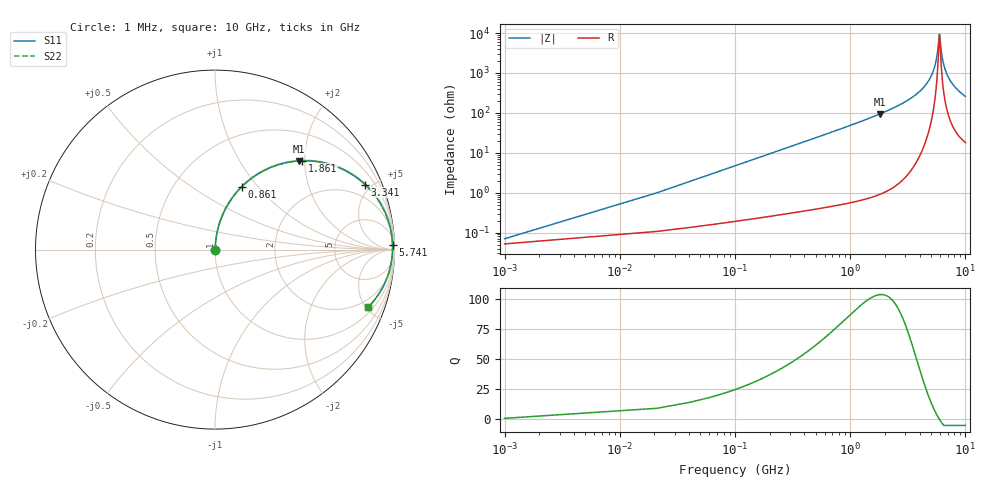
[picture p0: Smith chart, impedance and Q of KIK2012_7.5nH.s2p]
!version-2
!date-01.2022
!Series
# MHz S RI R 50
!Freq ReS11 ImS11 ReS21 ImS21 ReS12 ImS12 ReS22 ImS22
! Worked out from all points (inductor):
!   501 points, 1 MHz to 10 GHz, reference 50 ohm
!   read as one part in series: L = 7.5 nH near 41 MHz
!   highest Q = 103 at 1.801 GHz (marker M1), where L = 8.25 nH
!   self-resonance near 5.941 GHz
!   S11 on the Smith chart (normalised r, x): 1 MHz: 1.00, +0.00; 861 MHz: 1.01, +0.83; 1.861 GHz: 1.02, +1.94; 3.341 GHz: 1.07, +4.59; 5.741 GHz: 26, +66; 10 GHz: 1.36, -5.17
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1  0.000521 0.000471  0.9995 -0.000471  0.9995 -0.000471  0.000521 0.000471
61  0.00239 0.0286  0.9976 -0.0286  0.9976 -0.0286  0.00239 0.0286
101  0.00416 0.0473  0.9958 -0.0473  0.9958 -0.0473  0.00416 0.0473
181  0.00962 0.0843  0.9904 -0.0843  0.9904 -0.0843  0.00962 0.0843
301  0.0227 0.1386  0.9773 -0.1386  0.9773 -0.1386  0.0227 0.1386
441  0.045 0.1988  0.955 -0.1988  0.955 -0.1988  0.045 0.1988
861  0.1496 0.3506  0.8504 -0.3506  0.8504 -0.3506  0.1496 0.3506
1681  0.4263 0.4897  0.5737 -0.4897  0.5737 -0.4897  0.4263 0.4897
1801  0.4663 0.4941  0.5337 -0.4941  0.5337 -0.4941  0.4663 0.4941
1861  0.4859 0.495  0.5141 -0.495  0.5141 -0.495  0.4859 0.495
3341  0.8369 0.3619  0.1631 -0.3619  0.1631 -0.3619  0.8369 0.3619
4301  0.941 0.2206  0.059 -0.2206  0.059 -0.2206  0.941 0.2206
5001  0.9765 0.1213  0.0235 -0.1213  0.0235 -0.1213  0.9765 0.1213
5441  0.9865 0.0633  0.0135 -0.0633  0.0135 -0.0633  0.9865 0.0633
5741  0.9892 0.0259  0.0108 -0.0259  0.0108 -0.0259  0.9892 0.0259
5901  0.9894 0.00672  0.0106 -0.00672  0.0106 -0.00672  0.9894 0.00672
5961  0.9893 -0.000332  0.0107 0.000332  0.0107 0.000332  0.9893 -0.000332
6281  0.987 -0.0367  0.013 0.0367  0.013 0.0367  0.987 -0.0367
6681  0.9808 -0.0791  0.0192 0.0791  0.0192 0.0791  0.9808 -0.0791
7341  0.964 -0.142  0.036 0.142  0.036 0.142  0.964 -0.142
8341  0.928 -0.222  0.072 0.222  0.072 0.222  0.928 -0.222
10000  0.8539 -0.3199  0.1461 0.3199  0.1461 0.3199  0.8539 -0.3199
